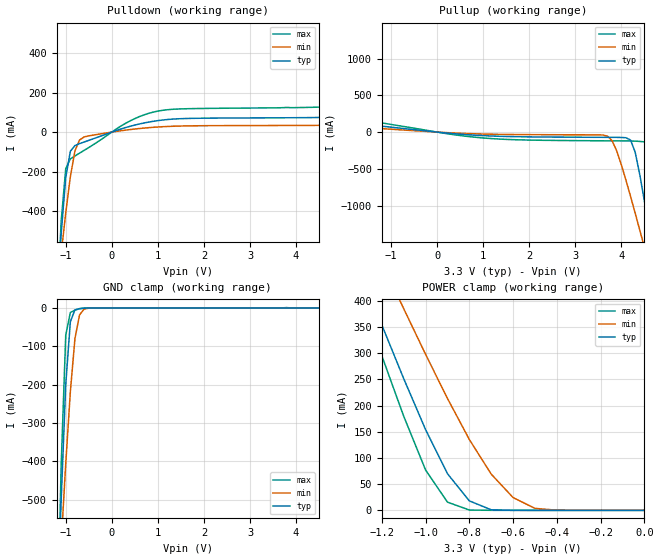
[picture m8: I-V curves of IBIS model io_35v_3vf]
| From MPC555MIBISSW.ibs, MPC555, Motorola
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| io_35v_3vf
[Model]   io_35v_3vf
Model_type   I/O
Polarity   Non-Inverting
|   typ   min   max
C_comp   7.9550e-13   7.1400e-13   9.0400e-13
| CAP models
| typical : model= typ
| maximum : model= wcs
| minimum : model= bcs
[Voltage range]   3.3v   3.0v   3.6v
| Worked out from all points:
|   slope of the pulldown table from 0 to 0.495 V, typ, clamps not added: 14 ohm
|   slope of the pullup table from 0 to 0.495 V, typ, clamps not added: 17.5 ohm
|   GND clamp passes 1 mA (typ) near -0.66 V on its own axis
|   POWER clamp passes 1 mA (typ) near -0.69 V on its own axis
|  typical: model = typ,  temp = 25,  vdd = 3.3
|  maximum: model = bcs,  temp = -40, vdd = 3.6
|  minimum: model = wcs,  temp = 150, vdd = 3.3
[Pulldown]
|  Voltage   I(typ)   I(min)   I(max)
-3.3V     -9.364A    -5.891A    -14.17A
-1.2V     -870.1mA   -838.4mA   -963.6mA
-1.1V     -518.6mA   -618.8mA   -455mA
-1V       -230.3mA   -410.8mA   -185mA
-900mV    -97.35mA   -226.4mA   -136mA
-600mV    -50.22mA   -24.44mA   -92.7mA
1.1V      61.12mA    27.2mA     110.4mA
5.5V      80.67mA    40.54mA    139.8mA
5.9V      156.1mA    252.8mA    165.8mA
6.2V      445.6mA    515.8mA    455.6mA
6.3V      552.9mA    607.1mA    579.4mA
6.6V      883.1mA    886.2mA    963.1mA
[GND_clamp]
-5V       -16.37A    -10.07A    -25.06A
-1.2V     -862.4mA   -836.3mA   -946.1mA
-1.1V     -505.3mA   -615.9mA   -414.3mA
-1V       -199.6mA   -406.4mA   -70.86mA
-900mV    -35.61mA   -218.7mA   -11.66mA
-800mV    -4.848mA   -79.69mA   -5.389mA
-700mV    -1.447mA   -17.89mA   -1.793mA
-600mV    -340.2uA   -2.494mA   -242uA
-500mV    -43.62uA   -353.5uA   -9.885uA
5V        119.7pA    22.38nA    107.4pA
[Pullup]
-3.3V     992mA      696.2mA    1.461A
-2.6V     239.7mA    127.9mA    543.2mA
-2.3V     151.6mA    91.46mA    240.2mA
3.6V      -71.02mA   -40.01mA   -118.5mA
3.8V      -71.48mA   -117.4mA   -119.2mA
4.1V      -76.87mA   -653.9mA   -120.3mA
4.3V      -272mA     -1.101A    -122.8mA
4.4V      -577.9mA   -1.333A    -126.7mA
4.6V      -1.313A    -1.803A    -192.9mA
4.7V      -1.701A    -2.04A     -536.7mA
4.9V      -2.494A    -2.519A    -1.653A
6.6V      -9.447A    -6.671A    -12.4A
[POWER_clamp]
-5V       4.559A     4.065A     5.11A
-1.3V     459.2mA    564.9mA    415.1mA
-1.2V     354.1mA    474.5mA    295.2mA
-1.1V     251.6mA    385.3mA    179.8mA
-1V       154.2mA    298mA      77.05mA
-900mV    70.04mA    213.8mA    15.71mA
-800mV    18.08mA    135.3mA    606.6uA
-700mV    1.079mA    69.19mA    104.9uA
-600mV    34.26uA    24.39mA    21.06uA
-500mV    2.117uA    3.8mA      1.676uA
-400mV    134.1nA    287.6uA    45.96nA
0V        119.7pA    21.86nA    118.6pA
| RAMP models
| typical dv/dt : model=typ, temp=25
| maximum dv/dt : model=bcs, temp=-40
| minimum dv/dt : model=wcs, temp=150
|		 typ   min   max
[Ramp]
dV/dt_r   1.52553/4.00435E-10   0.940967/4.47077E-10   2.23593/2.37562E-10
dV/dt_f   1.52553/3.46867E-10   0.940967/4.80319E-10   2.23593/2.12483E-10
